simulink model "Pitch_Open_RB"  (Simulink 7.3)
settings: Solver=ode45  StartTime=0.0  StopTime=20  RelTol=1e-3
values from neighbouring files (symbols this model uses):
  Aac = [    [actuator_srb.m]    (also in actuator_ssme.m; actuators_5s.m; actuators_5z.m)
  Bac = [    [actuator_srb.m]    (also in actuator_ssme.m; actuators_5s.m; actuators_5z.m)
  Cac = [    [actuator_srb.m]    (also in actuator_ssme.m; actuators_5s.m; actuators_5z.m)
  Dac = [    [actuator_srb.m]    (also in actuator_ssme.m; actuators_5s.m; actuators_5z.m)
undefined symbols (not defined in the file or in its folder): Afs, Apr, Asb, Bfs, Bpr, Bsb, Cfs, Cpr, Csb, Dfs, Dpr, Dsb

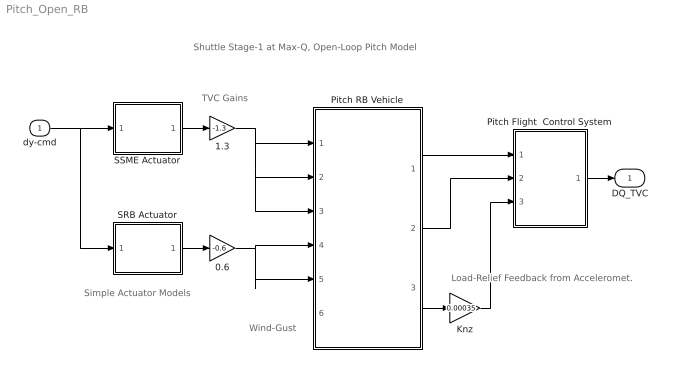
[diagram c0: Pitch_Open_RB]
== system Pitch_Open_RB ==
  note: TVC Gains
  note: Shuttle Stage-1 at Max-Q, Open-Loop Pitch Model
  note: Wind-Gust
  note: Load-Relief Feedback from Acceleromet.
  note: Simple Actuator Models
  dy-cmd : Inport  OutDataType=sfix(16)  OutScaling=2^0
  0.6 : Gain  Gain=-0.6  ParameterDataType=sfix(16)  ParameterScaling=2^0  OutDataType=sfix(16)  OutScaling=2^0
  1.3 : Gain  Gain=-1.3  ParameterDataType=sfix(16)  ParameterScaling=2^0  OutDataType=sfix(16)  OutScaling=2^0
  Knz : Gain  Gain=0.00035  ParameterDataType=sfix(16)  ParameterScaling=2^0  OutDataType=sfix(16)  OutScaling=2^0
  Pitch Flight  Control System : Subsystem
  Pitch RB Vehicle : Subsystem
  SRB Actuator : Subsystem
  SSME Actuator : Subsystem
  DQ_TVC : Outport  OutDataType=sfix(16)  OutScaling=2^0
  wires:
  SSME Actuator/1(dy) -> 1.3/1
  dy-cmd/1 -> SSME Actuator/1(dy-com), SRB Actuator/1(dy-com)
  1.3/1 -> Pitch RB Vehicle/1(dy1), Pitch RB Vehicle/2(dy2), Pitch RB Vehicle/3(dy3)
  0.6/1 -> Pitch RB Vehicle/4(dy4), Pitch RB Vehicle/5(dy5)
  Pitch RB Vehicle/1(theta) -> Pitch Flight  Control System/1(theta)
  Pitch RB Vehicle/2(q-rb) -> Pitch Flight  Control System/2(q)
  Pitch RB Vehicle/3(Nz) -> Knz/1
  Knz/1 -> Pitch Flight  Control System/3(Nz)
  SRB Actuator/1(dy) -> 0.6/1
  Pitch Flight  Control System/1(DQ_TVC) -> DQ_TVC/1

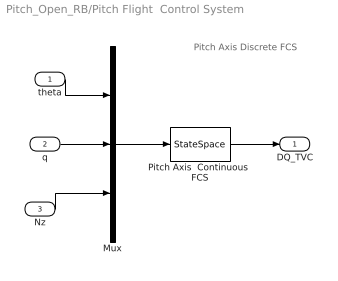
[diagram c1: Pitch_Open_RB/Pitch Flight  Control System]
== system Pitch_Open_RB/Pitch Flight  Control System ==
  note: Pitch Axis Discrete FCS
  theta : Inport  OutDataType=sfix(16)  OutScaling=2^0
  q : Inport  Port=2  OutDataType=sfix(16)  OutScaling=2^0
  Nz : Inport  Port=3  OutDataType=sfix(16)  OutScaling=2^0
  Mux : Mux  Inputs=3
  Pitch Axis  Continuous  FCS : StateSpace  A=Afs  B=Bfs  C=Cfs  D=Dfs
  DQ_TVC : Outport  OutDataType=sfix(16)  OutScaling=2^0
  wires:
  Pitch Axis  Continuous  FCS/1 -> DQ_TVC/1
  theta/1 -> Mux/1
  q/1 -> Mux/2
  Nz/1 -> Mux/3
  Mux/1 -> Pitch Axis  Continuous  FCS/1

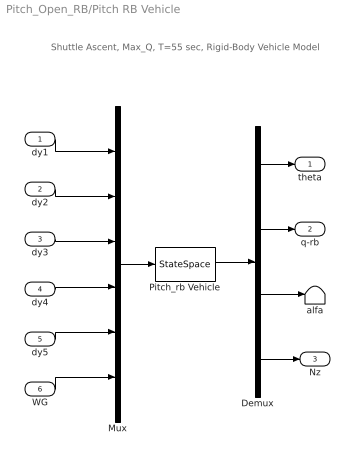
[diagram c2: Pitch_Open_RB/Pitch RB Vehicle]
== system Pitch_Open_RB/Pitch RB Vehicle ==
  note: Shuttle Ascent, Max_Q, T=55 sec, Rigid-Body Vehicle Model
  dy1 : Inport  OutDataType=sfix(16)  OutScaling=2^0
  dy2 : Inport  Port=2  OutDataType=sfix(16)  OutScaling=2^0
  dy3 : Inport  Port=3  OutDataType=sfix(16)  OutScaling=2^0
  dy4 : Inport  Port=4  OutDataType=sfix(16)  OutScaling=2^0
  dy5 : Inport  Port=5  OutDataType=sfix(16)  OutScaling=2^0
  WG : Inport  Port=6  OutDataType=sfix(16)  OutScaling=2^0
  Demux : Demux
  Mux : Mux  Inputs=6
  Pitch_rb Vehicle : StateSpace  A=Apr  B=Bpr  C=Cpr  D=Dpr
  alfa : Terminator
  theta : Outport  OutDataType=sfix(16)  OutScaling=2^0
  q-rb : Outport  Port=2  OutDataType=sfix(16)  OutScaling=2^0
  Nz : Outport  Port=3  OutDataType=sfix(16)  OutScaling=2^0
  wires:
  Pitch_rb Vehicle/1 -> Demux/1
  Mux/1 -> Pitch_rb Vehicle/1
  Demux/3 -> alfa/1
  dy1/1 -> Mux/1
  dy2/1 -> Mux/2
  dy3/1 -> Mux/3
  dy4/1 -> Mux/4
  dy5/1 -> Mux/5
  Demux/1 -> theta/1
  Demux/4 -> Nz/1
  Demux/2 -> q-rb/1
  WG/1 -> Mux/6

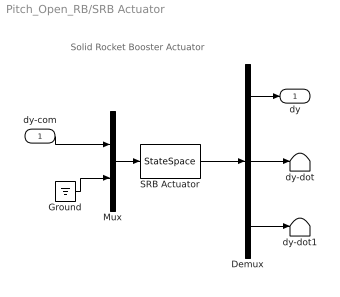
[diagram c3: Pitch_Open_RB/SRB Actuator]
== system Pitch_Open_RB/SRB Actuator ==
  note: Solid Rocket Booster Actuator
  dy-com : Inport  PortDimensions=1  OutDataType=sfix(16)  OutScaling=2^0
  Demux : Demux  Outputs=3
  Ground : Ground
  Mux : Mux  Inputs=2
  SRB Actuator : StateSpace  A=Asb  B=Bsb  C=Csb  D=Dsb
  dy-dot : Terminator
  dy-dot1 : Terminator
  dy : Outport  OutDataType=sfix(16)  OutScaling=2^0
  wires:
  SRB Actuator/1 -> Demux/1
  Mux/1 -> SRB Actuator/1
  Demux/1 -> dy/1
  Demux/2 -> dy-dot/1
  Demux/3 -> dy-dot1/1
  dy-com/1 -> Mux/1
  Ground/1 -> Mux/2

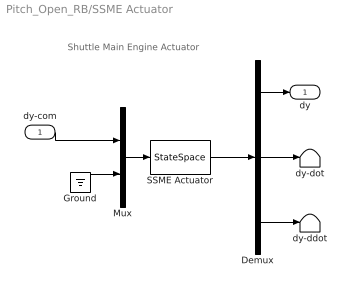
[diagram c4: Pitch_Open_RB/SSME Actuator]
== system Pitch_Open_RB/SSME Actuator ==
  note: Shuttle Main Engine Actuator
  dy-com : Inport  PortDimensions=1  OutDataType=sfix(16)  OutScaling=2^0
  Demux : Demux  Outputs=3
  Ground : Ground
  Mux : Mux  Inputs=2
  SSME Actuator : StateSpace  A=Aac  B=Bac  C=Cac  D=Dac
  dy-ddot : Terminator
  dy-dot : Terminator
  dy : Outport  OutDataType=sfix(16)  OutScaling=2^0
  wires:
  SSME Actuator/1 -> Demux/1
  Mux/1 -> SSME Actuator/1
  Demux/1 -> dy/1
  dy-com/1 -> Mux/1
  Demux/2 -> dy-dot/1
  Demux/3 -> dy-ddot/1
  Ground/1 -> Mux/2
